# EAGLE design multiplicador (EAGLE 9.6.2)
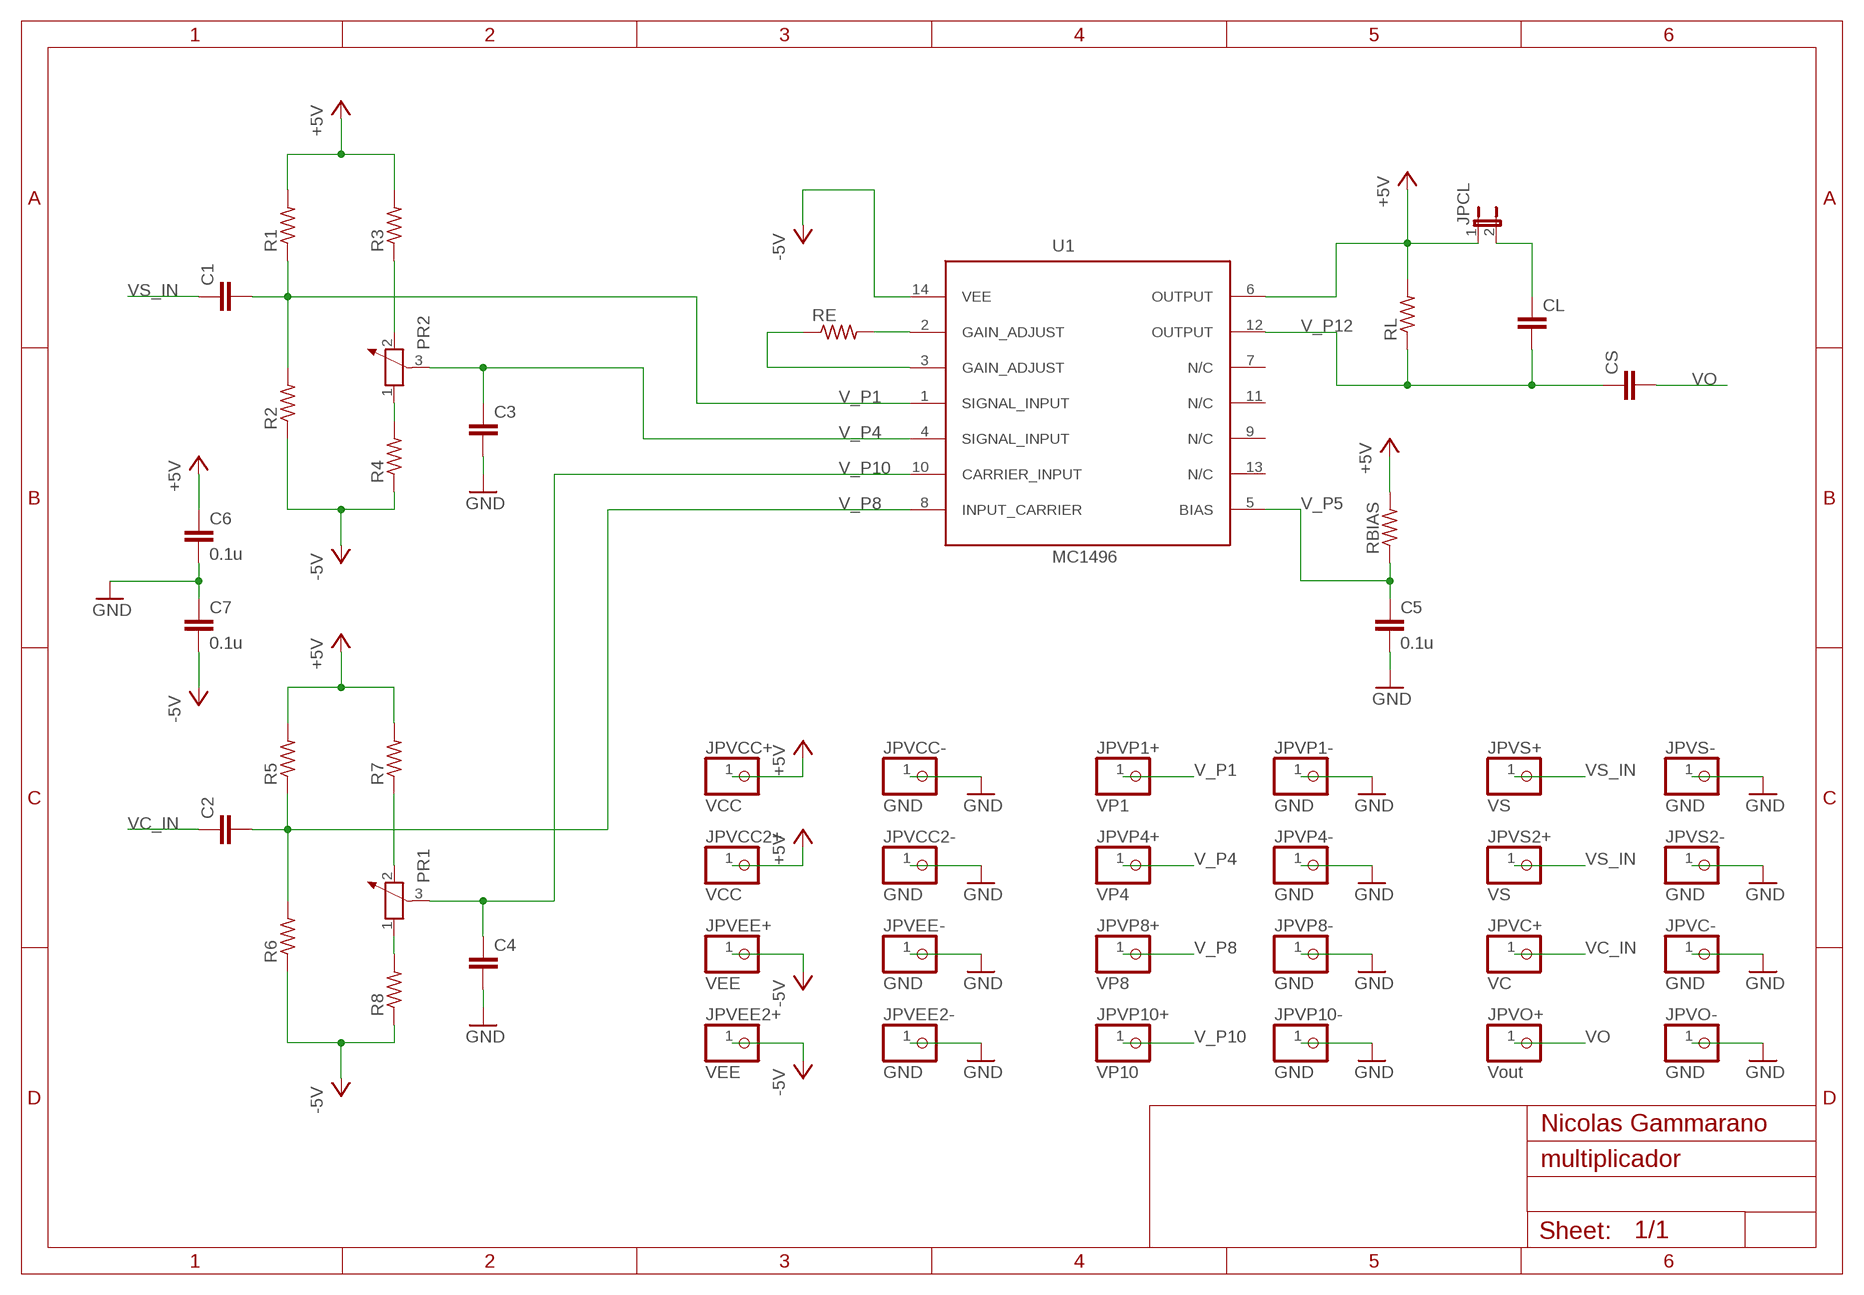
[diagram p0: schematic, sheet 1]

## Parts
C1  C-EU050-035X075  [C050-035X075]
C2  C-EU050-035X075  [C050-035X075]
C3  C-EU050-035X075  [C050-035X075]
C4  C-EU050-035X075  [C050-035X075]
C5  0.1u  C-EU050-035X075  [C050-035X075]
C6  0.1u  C-EU050-035X075  [C050-035X075]
C7  0.1u  C-EU050-035X075  [C050-035X075]
CL  C-EU050-035X075  [C050-035X075]
CS  C-EU050-035X075  [C050-035X075]
JPCL  JP1E  [JP1]
JPVC+  VC  PINHD-1X1  [1X01]
JPVC-  GND  PINHD-1X1  [1X01]
JPVCC2+  VCC  PINHD-1X1  [1X01]
JPVCC2-  GND  PINHD-1X1  [1X01]
JPVCC+  VCC  PINHD-1X1  [1X01]
JPVCC-  GND  PINHD-1X1  [1X01]
JPVEE2+  VEE  PINHD-1X1  [1X01]
JPVEE2-  GND  PINHD-1X1  [1X01]
JPVEE+  VEE  PINHD-1X1  [1X01]
JPVEE-  GND  PINHD-1X1  [1X01]
JPVO+  Vout  PINHD-1X1  [1X01]
JPVO-  GND  PINHD-1X1  [1X01]
JPVP1+  VP1  PINHD-1X1  [1X01]
JPVP1-  GND  PINHD-1X1  [1X01]
JPVP4+  VP4  PINHD-1X1  [1X01]
JPVP4-  GND  PINHD-1X1  [1X01]
JPVP8+  VP8  PINHD-1X1  [1X01]
JPVP8-  GND  PINHD-1X1  [1X01]
JPVP10+  VP10  PINHD-1X1  [1X01]
JPVP10-  GND  PINHD-1X1  [1X01]
JPVS2+  VS  PINHD-1X1  [1X01]
JPVS2-  GND  PINHD-1X1  [1X01]
JPVS+  VS  PINHD-1X1  [1X01]
JPVS-  GND  PINHD-1X1  [1X01]
PR1  POTENTIOMETER_PT_SPIN  [PT-SPIN]
PR2  POTENTIOMETER_PT_SPIN  [PT-SPIN]
R1  R-US_0207/10  [0207/10]
R2  R-US_0207/10  [0207/10]
R3  R-US_0207/10  [0207/10]
R4  R-US_0207/10  [0207/10]
R5  R-US_0207/10  [0207/10]
R6  R-US_0207/10  [0207/10]
R7  R-US_0207/10  [0207/10]
R8  R-US_0207/10  [0207/10]
RBIAS  R-US_0207/10  [0207/10]
RE  R-US_0207/10  [0207/10]
RL  R-US_0207/10  [0207/10]
U1  MC1496  [DIL14]

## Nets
+5V: C6.1 JPCL.1 JPVCC2+.1 JPVCC+.1 R1.2 R3.2 R5.2 R7.2 RBIAS.2 RL.2 U1.6(OUTPUT)
-5V: C7.2 JPVEE2+.1 JPVEE+.1 R2.1 R4.1 R6.1 R8.1 U1.14(VEE)
GND: C3.2 C4.2 C5.2 C6.2 C7.1 JPVC-.1 JPVCC2-.1 JPVCC-.1 JPVEE2-.1 JPVEE-.1 JPVO-.1 JPVP1-.1 JPVP4-.1 JPVP8-.1 JPVP10-.1 JPVS2-.1 JPVS-.1
N$4: PR2.2 R3.1
N$5: PR2.1 R4.2
N$6: RE.2 U1.2(GAIN_ADJUST)
N$7: RE.1 U1.3(GAIN_ADJUST)
N$10: PR1.1 R8.2
N$11: PR1.2 R7.1
N$15: CL.1 JPCL.2
V_P1: C1.2 JPVP1+.1 R1.1 R2.2 U1.1(SIGNAL_INPUT)
V_P4: C3.1 JPVP4+.1 PR2.3 U1.4(SIGNAL_INPUT)
V_P5: C5.1 RBIAS.1 U1.5(BIAS)
V_P8: C2.2 JPVP8+.1 R5.1 R6.2 U1.8(INPUT_CARRIER)
V_P10: C4.1 JPVP10+.1 PR1.3 U1.10(CARRIER_INPUT)
V_P12: CL.2 CS.1 RL.1 U1.12(OUTPUT)
VC_IN: C2.1 JPVC+.1
VO: CS.2 JPVO+.1
VS_IN: C1.1 JPVS2+.1 JPVS+.1
Unconnected: U1.7(N/C) U1.9(N/C) U1.11(N/C) U1.13(N/C)

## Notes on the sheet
- Nicolas Gammarano

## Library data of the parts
C1-C7 CL CS = rcl:C-EU: CAPACITOR, European symbol; SPICEPREFIX: C
JPCL = jumper:JP1E: JUMPER
JPVC+ JPVC- JPVCC2+ JPVCC2- JPVCC+ JPVCC- JPVEE2+ JPVEE2- JPVEE+ JPVEE- JPVO+ JPVO- JPVP1+ JPVP1- JPVP4+ JPVP4- JPVP8+ JPVP8- JPVP10+ JPVP10- JPVS2+ JPVS2- JPVS+ JPVS- = pinhead:PINHD-1X1: PIN HEADER
PR1 PR2 = rcl:POTENTIOMETER_: Potentiometer; SPICEMODEL: POT; SPICEPREFIX: X
R1-R8 RBIAS RE RL = rcl:R-US_: RESISTOR, American symbol; SPICEPREFIX: R
U1 = MC1496:MC1496: MC1496 MC1496 Balanced Modulators/Demodulators Source: https://www.onsemi.com/pub/Collateral/MC1496-D.PDF

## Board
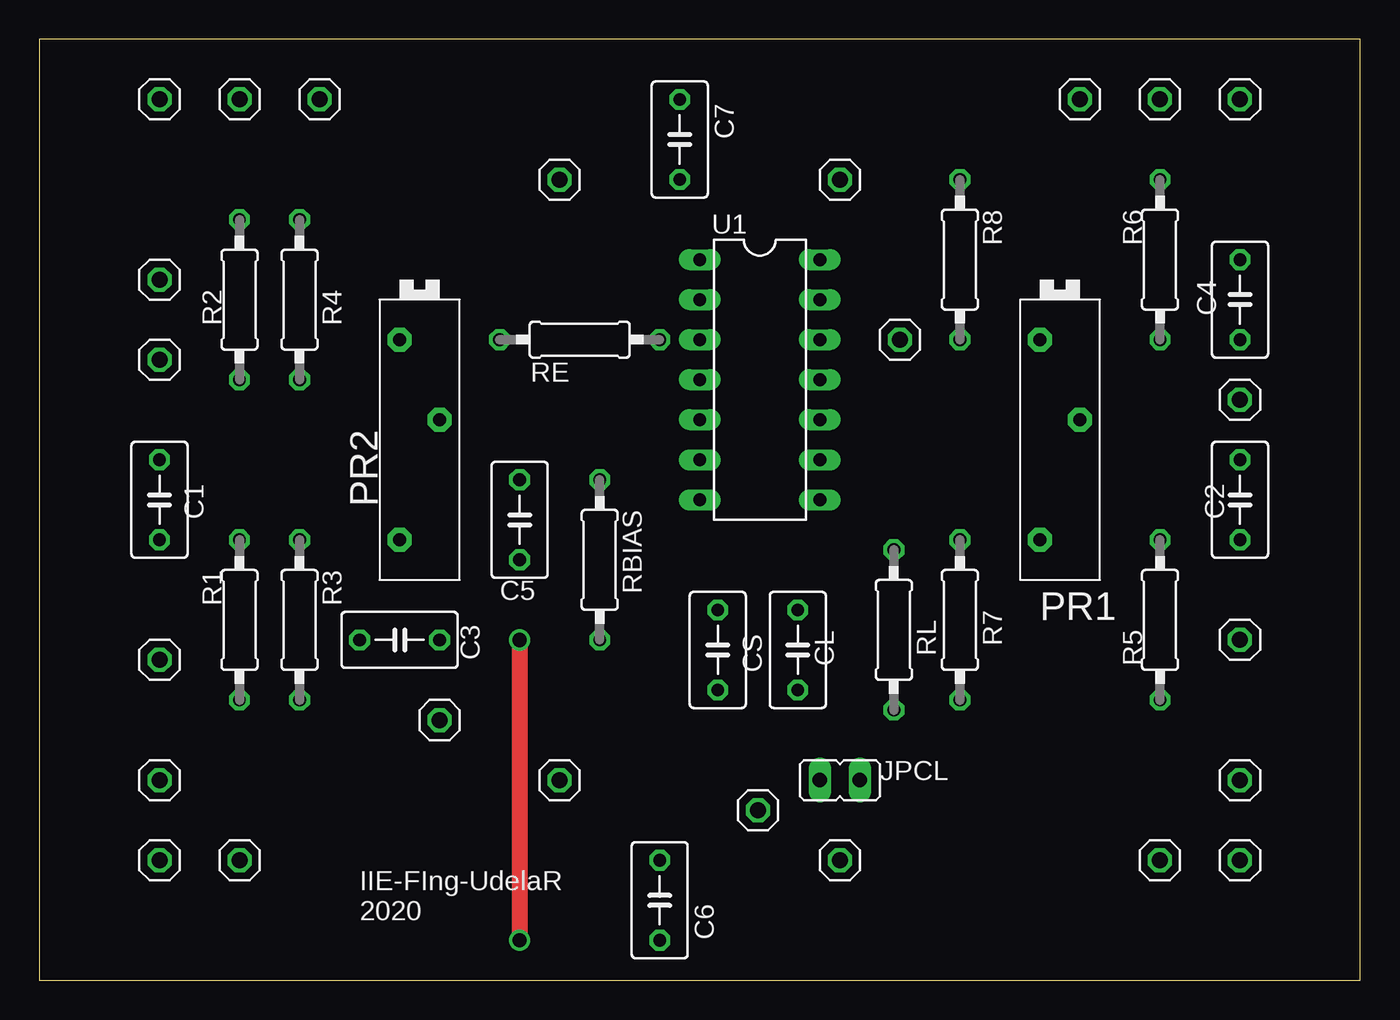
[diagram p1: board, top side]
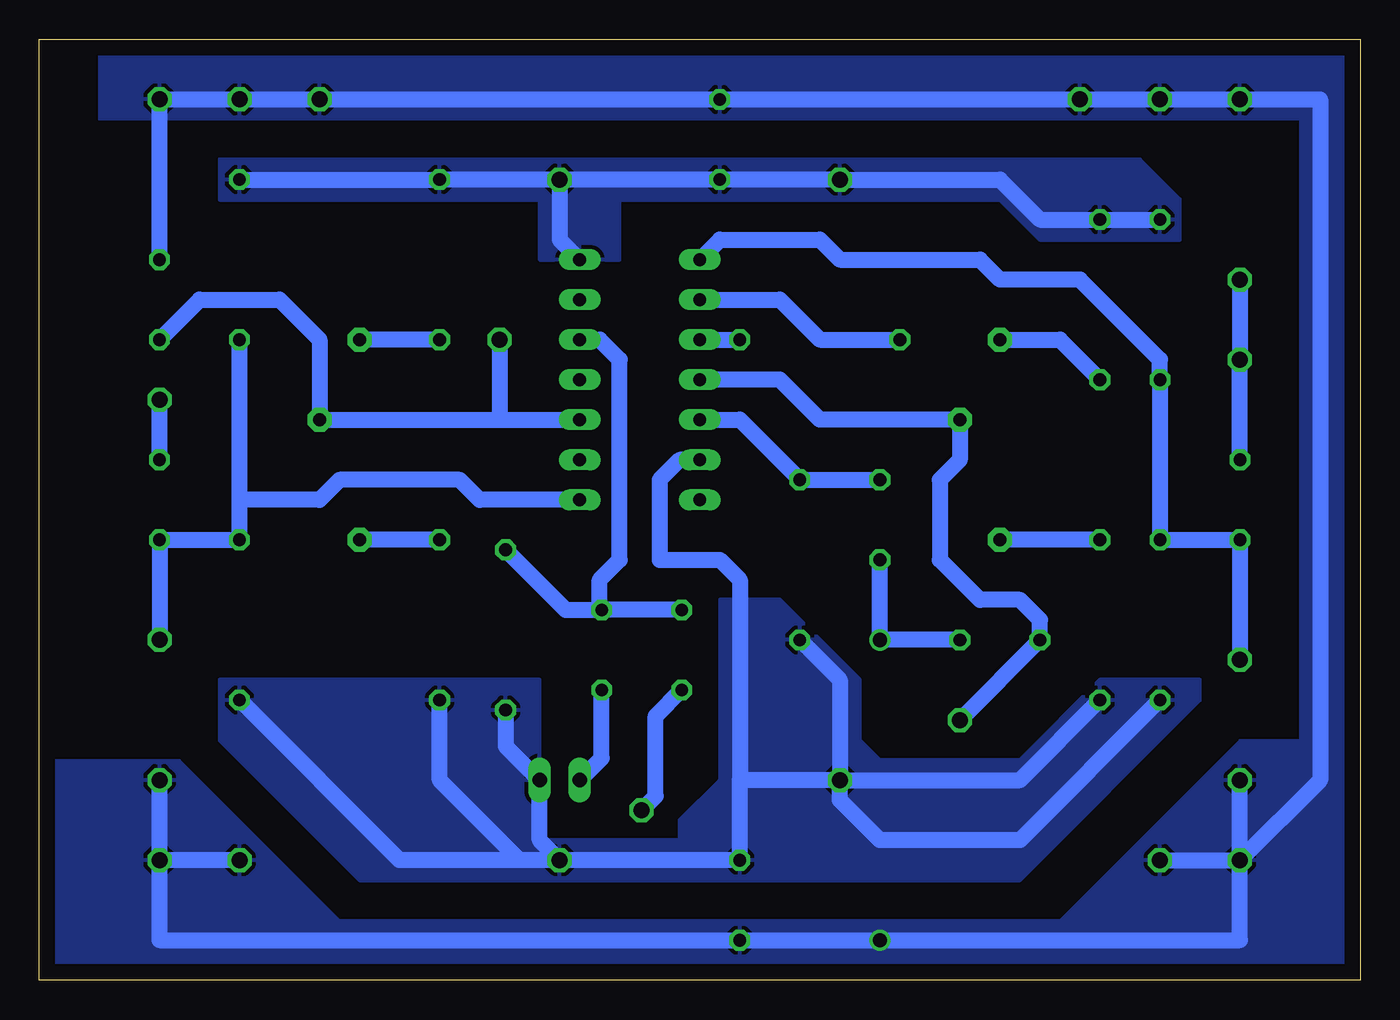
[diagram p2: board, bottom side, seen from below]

Size 83.82 x 59.69 mm. Coordinates in mm from the lower left corner, seen from the top.
Outline: 0,0 83.82,0 83.82,59.69 0,59.69 0,0
Copper layers (1*16): Top 0.035mm / dielectric 1.5mm / Bottom 0.035mm
Design rules "default": minimum track width 6mil, minimum drill 0.35mm, track to track 6mil, track to pad 6mil, pad to pad 6mil, via to via 6mil, smd to smd 6mil, copper to edge 40mil, drill to drill 6mil, minimum pad ring 10mil, minimum via ring 8mil, stop-mask expansion 4mil, vias tented up to drill 0mil, thermal gap 10mil

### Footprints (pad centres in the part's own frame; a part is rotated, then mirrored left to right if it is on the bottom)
C050-035X075 = drill 0.813 octagon: 1 -2.54,0; 2 2.54,0
JP1 = drill 0.914 long: 1 0,-1.27; 2 0,1.27
1X01 = drill 1.016 octagon: 1 0,0
PT-SPIN = drill 0.813 pad 1.524 octagon: 1 -6.35,-1.27; 2 6.35,-1.27; 3 -1.27,1.27
0207/10 = drill 0.813 octagon: 1 -5.08,0; 2 5.08,0
DIL14 = drill 0.813 long: 1 -7.62,-3.81; 2 -5.08,-3.81; 3 -2.54,-3.81; 4 0,-3.81; 5 2.54,-3.81; 6 5.08,-3.81; 7 7.62,-3.81; 8 7.62,3.81; 9 5.08,3.81; 10 2.54,3.81; 11 0,3.81; 12 -2.54,3.81; 13 -5.08,3.81; 14 -7.62,3.81

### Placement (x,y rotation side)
C1  7.62,30.48 270 top
C2  76.2,30.48 270 top
C3  22.86,21.59 0 top
C4  76.2,43.18 90 top
C5  30.48,29.21 270 top
C6  39.37,5.08 270 top
C7  40.64,53.34 270 top
CL  48.13,20.95 90 top
CS  43.05,20.95 270 top
JPCL  50.8,12.7 90 top
JPVC+  76.2,36.83 180 top
JPVC-  76.2,12.7 0 top
JPVCC2+  33.02,12.7 0 top
JPVCC2-  7.62,7.62 0 top
JPVCC+  50.8,7.62 0 top
JPVCC-  7.62,12.7 0 top
JPVEE2+  50.8,50.8 0 top
JPVEE2-  71.12,7.62 0 top
JPVEE+  33.02,50.8 0 top
JPVEE-  12.7,55.88 0 top
JPVO+  45.59,10.79 270 top
JPVO-  66.04,55.88 0 top
JPVP1+  7.62,20.32 0 top
JPVP1-  76.2,55.88 0 top
JPVP4+  25.4,16.51 0 top
JPVP4-  76.2,7.62 0 top
JPVP8+  76.2,21.59 0 top
JPVP8-  7.62,55.88 0 top
JPVP10+  54.61,40.64 0 top
JPVP10-  71.12,55.88 0 top
JPVS2+  7.62,44.45 0 top
JPVS2-  12.7,7.62 0 top
JPVS+  7.62,39.37 0 top
JPVS-  17.78,55.88 0 top
PR1  64.77,34.29 270 top
PR2  24.13,34.29 270 top
R1  12.7,22.86 270 top
R2  12.7,43.18 270 top
R3  16.51,22.86 270 top
R4  16.51,43.18 270 top
R5  71.12,22.86 270 top
R6  71.12,45.72 270 top
R7  58.42,22.86 270 top
R8  58.42,45.72 270 top
RBIAS  35.56,26.67 270 top
RE  34.29,40.64 180 top
RL  54.23,22.22 270 top
U1  45.72,38.1 270 top

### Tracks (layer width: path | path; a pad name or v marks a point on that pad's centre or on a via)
+5V
  Bottom 1.016: U1.6 43.18,33.02 44.45,31.75 44.45,26.67 40.64,26.67 39.37,25.4 39.37,12.7 | R1.2 21.59,8.89 30.48,8.89 33.02,11.43 JPVCC2+.1 | JPVCC2+.1 21.59,12.7 R3.2 | RBIAS.2 33.02,19.05 JPVCC2+.1 | JPVCC2+.1 39.37,12.7 | JPVCC+.1 C6.1 39.37,12.7 | JPVCC+.1 53.34,7.62 58.42,12.7 R7.2 | R5.2 60.96,7.62 JPVCC+.1 | RL.2 54.23,14.86 JPCL.1 52.07,8.89 JPVCC+.1
  pour Bottom (isolate 0.406): 10.16,19.05 16.51,19.05 21.59,13.97 30.48,13.97 31.75,15.24 31.75,19.05 36.83,24.13 40.64,24.13 40.64,12.7 43.18,10.16 43.18,8.89 52.07,8.89 52.07,19.05 72.39,19.05 72.39,15.24 63.5,6.35 21.59,6.35 10.16,17.78
-5V
  Bottom 1.016: JPVEE2+.1 50.8,46.99 U1.14 | JPVEE2+.1 R8.1 R6.1 | JPVEE2+.1 C7.2 JPVEE+.1 22.86,50.8 20.32,48.26 R4.1 R2.1
  pour Bottom (isolate 0.406): 11.43,49.53 13.97,52.07 72.39,52.07 72.39,49.53 52.07,49.53 52.07,45.72 46.99,45.72 46.99,49.53 22.86,49.53 20.32,46.99 11.43,46.99
GND  (via drill 0.9, 0.9 pad 0.9)
  Top 1.016: v30.48,21.59 v30.48,2.54
  Bottom 1.016: JPVCC2-.1 7.62,2.54 v30.48,2.54 C6.2 76.2,2.54 JPVP4-.1 | JPVCC2-.1 JPVCC-.1 | JPVS2-.1 JPVCC2-.1 | JPVEE2-.1 JPVP4-.1 | JPVP4-.1 JPVC-.1 | C4.2 JPVP1-.1 JPVP10-.1 JPVP8-.1 2.54,55.88 2.54,12.7 JPVCC2-.1 | C3.2 v30.48,21.59 C5.2
  pour Bottom: 3.81,54.61 80.01,54.61 80.01,59.69 0,59.69 0,0 83.82,0 83.82,13.97 74.93,13.97 64.77,3.81 19.05,3.81 7.62,15.24 3.81,15.24
N$4
  Bottom 1.016: R3.1 PR2.2
N$5
  Bottom 1.016: PR2.1 19.05,40.64 R4.2
N$6
  Bottom 1.016: U1.2 36.83,43.18 34.29,40.64 RE.2
N$7
  Bottom 1.016: U1.3 RE.1
N$10
  Bottom 1.016: R8.2 PR1.1
N$11
  Bottom 1.016: R7.1 PR1.2
N$15
  Bottom 1.016: CL.1 48.13,14.1 JPCL.2
V_P1
  Bottom 1.016: JPVP1+.1 C1.2 R1.1 R2.2 12.7,39.37 17.78,44.45 22.86,44.45 24.13,45.72 33.02,45.72 34.29,46.99 40.64,46.99 U1.1
V_P4
  Bottom 1.016: U1.4 36.83,38.1 34.29,35.56 PR2.3 25.4,33.02 26.67,31.75 26.67,26.67 24.13,24.13 21.59,24.13 20.32,22.86 C3.1 JPVP4+.1
V_P5
  Bottom 1.016: U1.5 39.37,35.56 RBIAS.1 C5.1
V_P8
  Bottom 1.016: 71.12,30.48 R5.1 C2.2 JPVP8+.1 | 71.12,30.48 R6.2 | U1.8 55.88,30.48 57.15,31.75 64.77,31.75 66.04,30.48 71.12,30.48
V_P10
  Bottom 1.016: 54.61,35.56 PR1.3 66.04,40.64 68.58,43.18 73.66,43.18 C4.1 | 54.61,35.56 U1.10 | JPVP10+.1 54.61,35.56
V_P12
  Bottom 1.016: U1.12 48.26,40.64 46.99,39.37 46.99,26.67 48.26,25.4 48.26,23.62 CL.2 | RL.1 50.42,23.5 CL.2 | CS.1 CL.2
VC_IN
  Bottom 1.016: C2.1 JPVC+.1
VO
  Bottom 1.016: CS.2 44.7,16.76 44.7,11.68 JPVO+.1
VS_IN
  Bottom 1.016: C1.1 JPVS+.1 JPVS2+.1

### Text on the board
tNames: IIE-FIng-UdelaR / 2020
